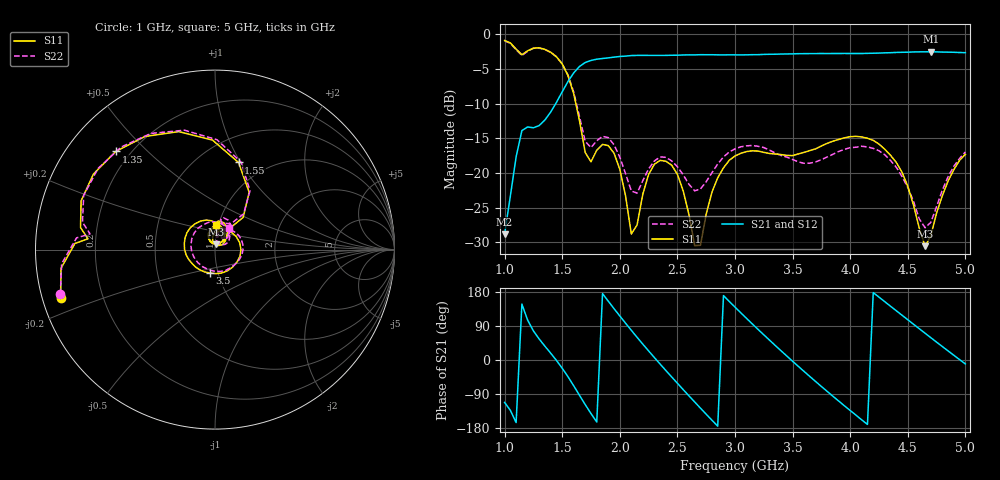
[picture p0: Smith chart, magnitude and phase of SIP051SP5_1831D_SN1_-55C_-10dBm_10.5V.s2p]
# GHz  S  dB  R  50
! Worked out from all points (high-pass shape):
!   81 points, 1 GHz to 5 GHz, reference 50 ohm
!   highest |S21| = -2.54 dB at 4.7 GHz (marker M1); lowest = -28.8 dB at 1 GHz (marker M2)
!   |S21| within 3 dB of the highest: 1.602 GHz to end of sweep
!   lowest |S11| = -30.5 dB at 4.65 GHz (marker M3), VSWR 1.06, Z = 50.6 + j2.93 ohm
!   |S11| at or under -10 dB: 1.618 GHz to end of sweep
!   |S22| runs from -27.9 to -0.9 dB; largest |S21 - S12| = 0.0022
!   S11 on the Smith chart (normalised r, x): 1 GHz: 0.05, -0.15; 1.35 GHz: 0.15, +0.40; 1.55 GHz: 0.75, +0.98; 3.5 GHz: 0.91, -0.24; 5 GHz: 0.97, +0.27
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1  -0.90 -162.5  -28.81 -111.9  -28.84 -111.9  -0.94 -163.9
1.15  -2.97 175.2  -13.89 147.5  -13.90 147.6  -3.08 172.8
1.35  -2.18 135.3  -12.36 36.4  -12.38 36.4  -2.22 132.5
1.55  -5.97 74.9  -6.83 -44.0  -6.83 -44.0  -5.87 73.4
1.7  -17.06 55.8  -4.08 -117.8  -4.08 -117.8  -15.44 58.4
1.85  -15.88 83.4  -3.50 175.3  -3.50 175.3  -14.72 74.9
2.05  -23.30 45.4  -3.16 97.1  -3.15 97.2  -20.10 47.2
2.1  -28.79 64.8  -3.08 78.4  -3.08 78.4  -22.59 57.8
2.35  -18.18 88.5  -3.06 -10.8  -3.05 -10.7  -17.68 71.3
2.5  -20.19 49.8  -3.03 -61.4  -3.03 -61.4  -19.09 47.6
2.65  -30.46 48.5  -2.98 -110.8  -2.97 -110.8  -22.56 52.2
2.85  -20.68 89.0  -2.98 -174.6  -2.97 -174.6  -18.70 63.0
3  -17.55 46.6  -2.98 139.6  -2.97 139.5  -16.53 39.6
3.25  -17.03 -30.0  -2.91 66.5  -2.92 66.5  -16.33 -11.4
3.5  -17.49 -102.2  -2.84 -3.3  -2.83 -3.3  -18.05 -76.7
3.7  -16.52 -148.7  -2.79 -56.8  -2.79 -56.7  -18.41 -143.2
3.85  -15.42 179.7  -2.79 -95.6  -2.77 -95.6  -17.30 169.7
4.05  -14.71 138.1  -2.79 -145.6  -2.78 -145.7  -16.28 115.1
4.35  -17.44 76.2  -2.67 141.9  -2.68 141.9  -18.19 50.3
4.65  -30.54 76.6  -2.54 70.7  -2.55 70.6  -27.89 55.0
4.7  -29.05 109.1  -2.54 58.9  -2.55 58.9  -27.11 74.5
5  -17.32 88.4  -2.66 -10.4  -2.67 -10.4  -16.96 56.8
